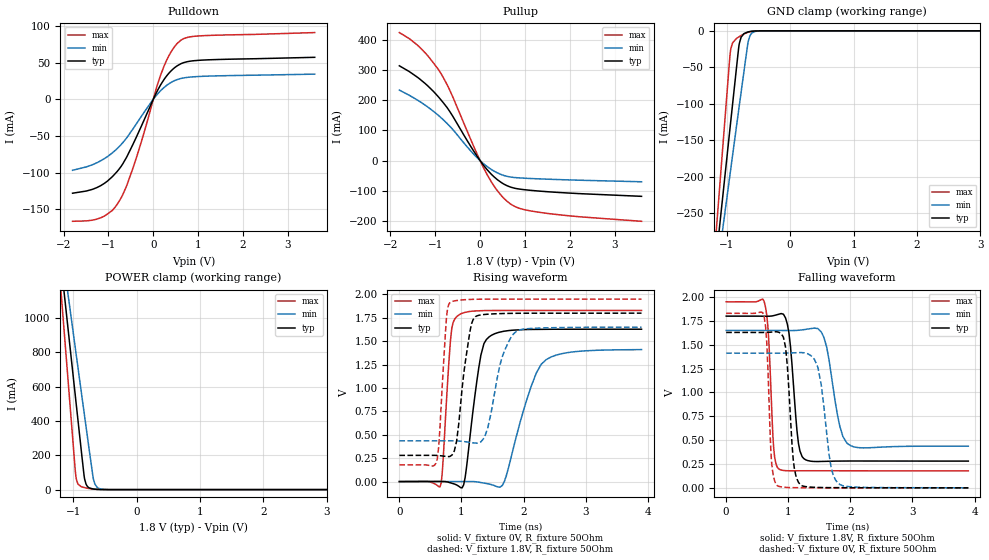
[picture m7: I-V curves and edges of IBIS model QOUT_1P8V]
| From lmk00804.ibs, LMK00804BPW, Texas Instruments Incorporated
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|   Model QOUT 1.8VCC
[Model]   QOUT_1P8V
Model_type   3-state
Polarity   Non-Inverting
Vmeas = 0.9
Vref = 1.8
Cref = 15pF
Rref = 50
|   typ   min   max
|   (fast PVT)   (slow PVT)   (nom PVT)
C_comp   0.315p   0.300p   0.317p
|C_comp (Hi state)   0.315p   0.300p   0.317p
|C_comp (Low state)   0.358p   0.325p   0.360p
[Voltage Range]   1.8   1.65   1.95
[Temperature Range]   45   125   -40
[Pullup Reference]   1.8   1.65   1.95
[Pulldown Reference]   -0   0   -0
[Power Clamp Reference]   1.8   1.65   1.95
[GND Clamp Reference]   0   0   0
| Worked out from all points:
|   slope of the pulldown table from 0 to 0.27 V, typ, clamps not added: 9.13 ohm
|   slope of the pullup table from 0 to 0.27 V, typ, clamps not added: 5.6 ohm
|   GND clamp passes 1 mA (typ) near -0.64 V on its own axis
|   POWER clamp passes 1 mA (typ) near -0.60 V on its own axis
|   falling waveform, V_fixture 1.8V, R_fixture 50Ohm: 20-80 % time 110ps typ, 182ps min, 72.7ps max; typ from 1.8 V to 0.281 V
|   rising waveform, V_fixture 0V, R_fixture 50Ohm: 20-80 % time 189ps typ, 379ps min, 102ps max; typ from 0 V to 1.63 V
|   rising waveform, V_fixture 1.8V, R_fixture 50Ohm: 20-80 % time 161ps typ, 241ps min, 92.8ps max; typ from 0.28 V to 1.8 V
|   falling waveform, V_fixture 0V, R_fixture 50Ohm: 20-80 % time 94.7ps typ, 157ps min, 64ps max; typ from 1.63 V to 0 V
[Pulldown]
|   Voltage   I(typ)   I(min)   I(max)
-1.8V     -128.1mA   -96.87mA   -166.5mA
-1.174V   -117.9mA   -83.94mA   -161.8mA
-914.4mV  -105.7mA   -73.2mA    -151.6mA
-725.4mV  -92.26mA   -62.34mA   -135.4mA
-579.6mV  -77.22mA   -51.51mA   -115.7mA
-369mV    -50.49mA   -32.71mA   -78.23mA
52.2mV    6.895mA    4.125mA    11.61mA
171mV     20.43mA    12.22mA    34.26mA
387mV     38.15mA    22.66mA    63.7mA
613.8mV   48.46mA    28.38mA    80.54mA
1.067V    53.39mA    31.27mA    86.66mA
3.6V      57.3mA     34.32mA    91.07mA
[GND Clamp]
|   Voltage   I(typ)   I(min)   I(max)
-1.8V     -835mA     -756.1mA   -984.2mA
-1.163V   -308.5mA   -336mA     -270.7mA
-1.103V   -259.7mA   -297.2mA   -204.5mA
-957.6mV  -140.6mA   -202.4mA   -42.25mA
-936mV    -123mA     -188.4mA   -24.65mA
-909mV    -101.1mA   -170.9mA   -16.53mA
-806.4mV  -19.71mA   -105mA     -8.165mA
-774mV    -8.809mA   -84.29mA   -6.451mA
-725.4mV  -3.676mA   -53.43mA   -4.191mA
-655.2mV  -1.35mA    -12.48mA   -1.766mA
-552.6mV  -217.2uA   -777.4uA   -243uA
3.6V      0A         0A         0A
[Pullup]
|   Voltage   I(typ)   I(min)   I(max)
-1.8V     315mA      234.2mA    425.4mA
-1.346V   271.2mA    196.4mA    376.7mA
-1.163V   247.8mA    177.7mA    347.7mA
-903.6mV  207.3mA    146.9mA    296.8mA
-676.8mV  163.2mA    114.4mA    234.1mA
-163.8mV  36.67mA    24.8mA     54.64mA
84.6mV    -17.01mA   -11.18mA   -26.08mA
376.2mV   -62.31mA   -40.11mA   -98.25mA
613.8mV   -84.22mA   -52.77mA   -136.7mA
862.2mV   -94.28mA   -57.38mA   -157.9mA
1.294V    -101mA     -60.56mA   -171.2mA
3.6V      -118.7mA   -70.39mA   -201.7mA
[POWER Clamp]
|   Voltage   I(typ)   I(min)   I(max)
-1.8V     3.418A     3.118A     4.01A
-1.233V   1.46A      1.554A     1.349A
-1.152V   1.182A     1.332A     971.3mA
-979.2mV  592.7mA    861.3mA    169.7mA
-957.6mV  519.3mA    802.6mA    80.2mA
-925.2mV  409.3mA    714.7mA    33.06mA
-876.6mV  244.7mA    583mA      17.91mA
-828mV    82.92mA    451.6mA    12.36mA
-795.6mV  31.2mA     364.1mA    9.555mA
-682.2mV  3.593mA    65.43mA    2.774mA
-558mV    452.5uA    2.383mA    294.6uA
3.6V      0A         0A         0A
[Ramp]
R_load = 50
|   typ   min   max
dV/dt_r   0.97706/1.89201e-10   0.846114/3.78689e-10   1.09721/1.01693e-10
dV/dt_f   0.911662/1.09511e-10   0.727837/1.81689e-10   1.06298/7.26782e-11
[Falling Waveform]
V_fixture = 1.8V
V_fixture_min = 1.65V
V_fixture_max = 1.95V
R_fixture = 50Ohm
C_fixture = 0F
|   Time   V(typ)   V(min)   V(max)
0s        1.8V       1.65V      1.95V
610.6ps   1.799V     1.65V      1.955V
672.8ps   1.799V     1.65V      1.682V
766.8ps   1.806V     1.65V      405.4mV
844.3ps   1.819V     1.65V      199.7mV
1.011ns   1.625V     1.649V     179.3mV
1.25ns    307.3mV    1.658V     179.6mV
1.573ns   277.7mV    1.578V     179.6mV
1.947ns   281.5mV    467.4mV    179.2mV
3.9ns     280.6mV    436.9mV    178.4mV
[Rising Waveform]
V_fixture = 0V
V_fixture_min = 0V
V_fixture_max = 0V
R_fixture = 50Ohm
C_fixture = 0F
|   Time   V(typ)   V(min)   V(max)
0s        446.5pV    16.61nV    376.6pV
653.1ps   1.407mV    189.4uV    -56.92mV
844.3ps   -17.78mV   244.8uV    1.638V
962.1ps   -52.57mV   278.9uV    1.782V
1.059ns   43.8mV     307.2uV    1.809V
1.313ns   1.351V     -10.35mV   1.826V
1.446ns   1.547V     -26.61mV   1.828V
1.691ns   1.607V     2.009mV    1.828V
2.364ns   1.627V     1.303V     1.829V
3.9ns     1.628V     1.41V      1.829V
[Rising Waveform]
V_fixture = 1.8V
V_fixture_min = 1.65V
V_fixture_max = 1.95V
R_fixture = 50Ohm
C_fixture = 0F
|   Time   V(typ)   V(min)   V(max)
0s        279.8mV    435.3mV    178mV
589.1ps   279.8mV    435.4mV    197mV
634.3ps   277.5mV    435.5mV    374.5mV
755.6ps   268mV      436mV      1.722V
824.5ps   273.3mV    436mV      1.918V
921.5ps   429.9mV    434.7mV    1.935V
1.079ns   1.355V     423.9mV    1.945V
1.224ns   1.762V     411.9mV    1.948V
1.881ns   1.798V     1.603V     1.95V
3.9ns     1.8V       1.649V     1.95V
[Falling Waveform]
|Gnd
V_fixture = 0V
V_fixture_min = 0V
V_fixture_max = 0V
R_fixture = 50Ohm
C_fixture = 0F
|   Time   V(typ)   V(min)   V(max)
0s        1.629V     1.412V     1.829V
610.6ps   1.629V     1.412V     1.798V
730.6ps   1.633V     1.412V     274.8mV
824.5ps   1.634V     1.412V     22.46mV
956.2ps   1.474V     1.413V     5.688mV
1.079ns   298.9mV    1.415V     2.671mV
1.188ns   37.43mV    1.418V     1.866mV
1.477ns   4.766mV    1.264V     1.482mV
1.833ns   2.236mV    34.63mV    1.012mV
3.9ns     493.4uV    1.001mV    283.9uV
